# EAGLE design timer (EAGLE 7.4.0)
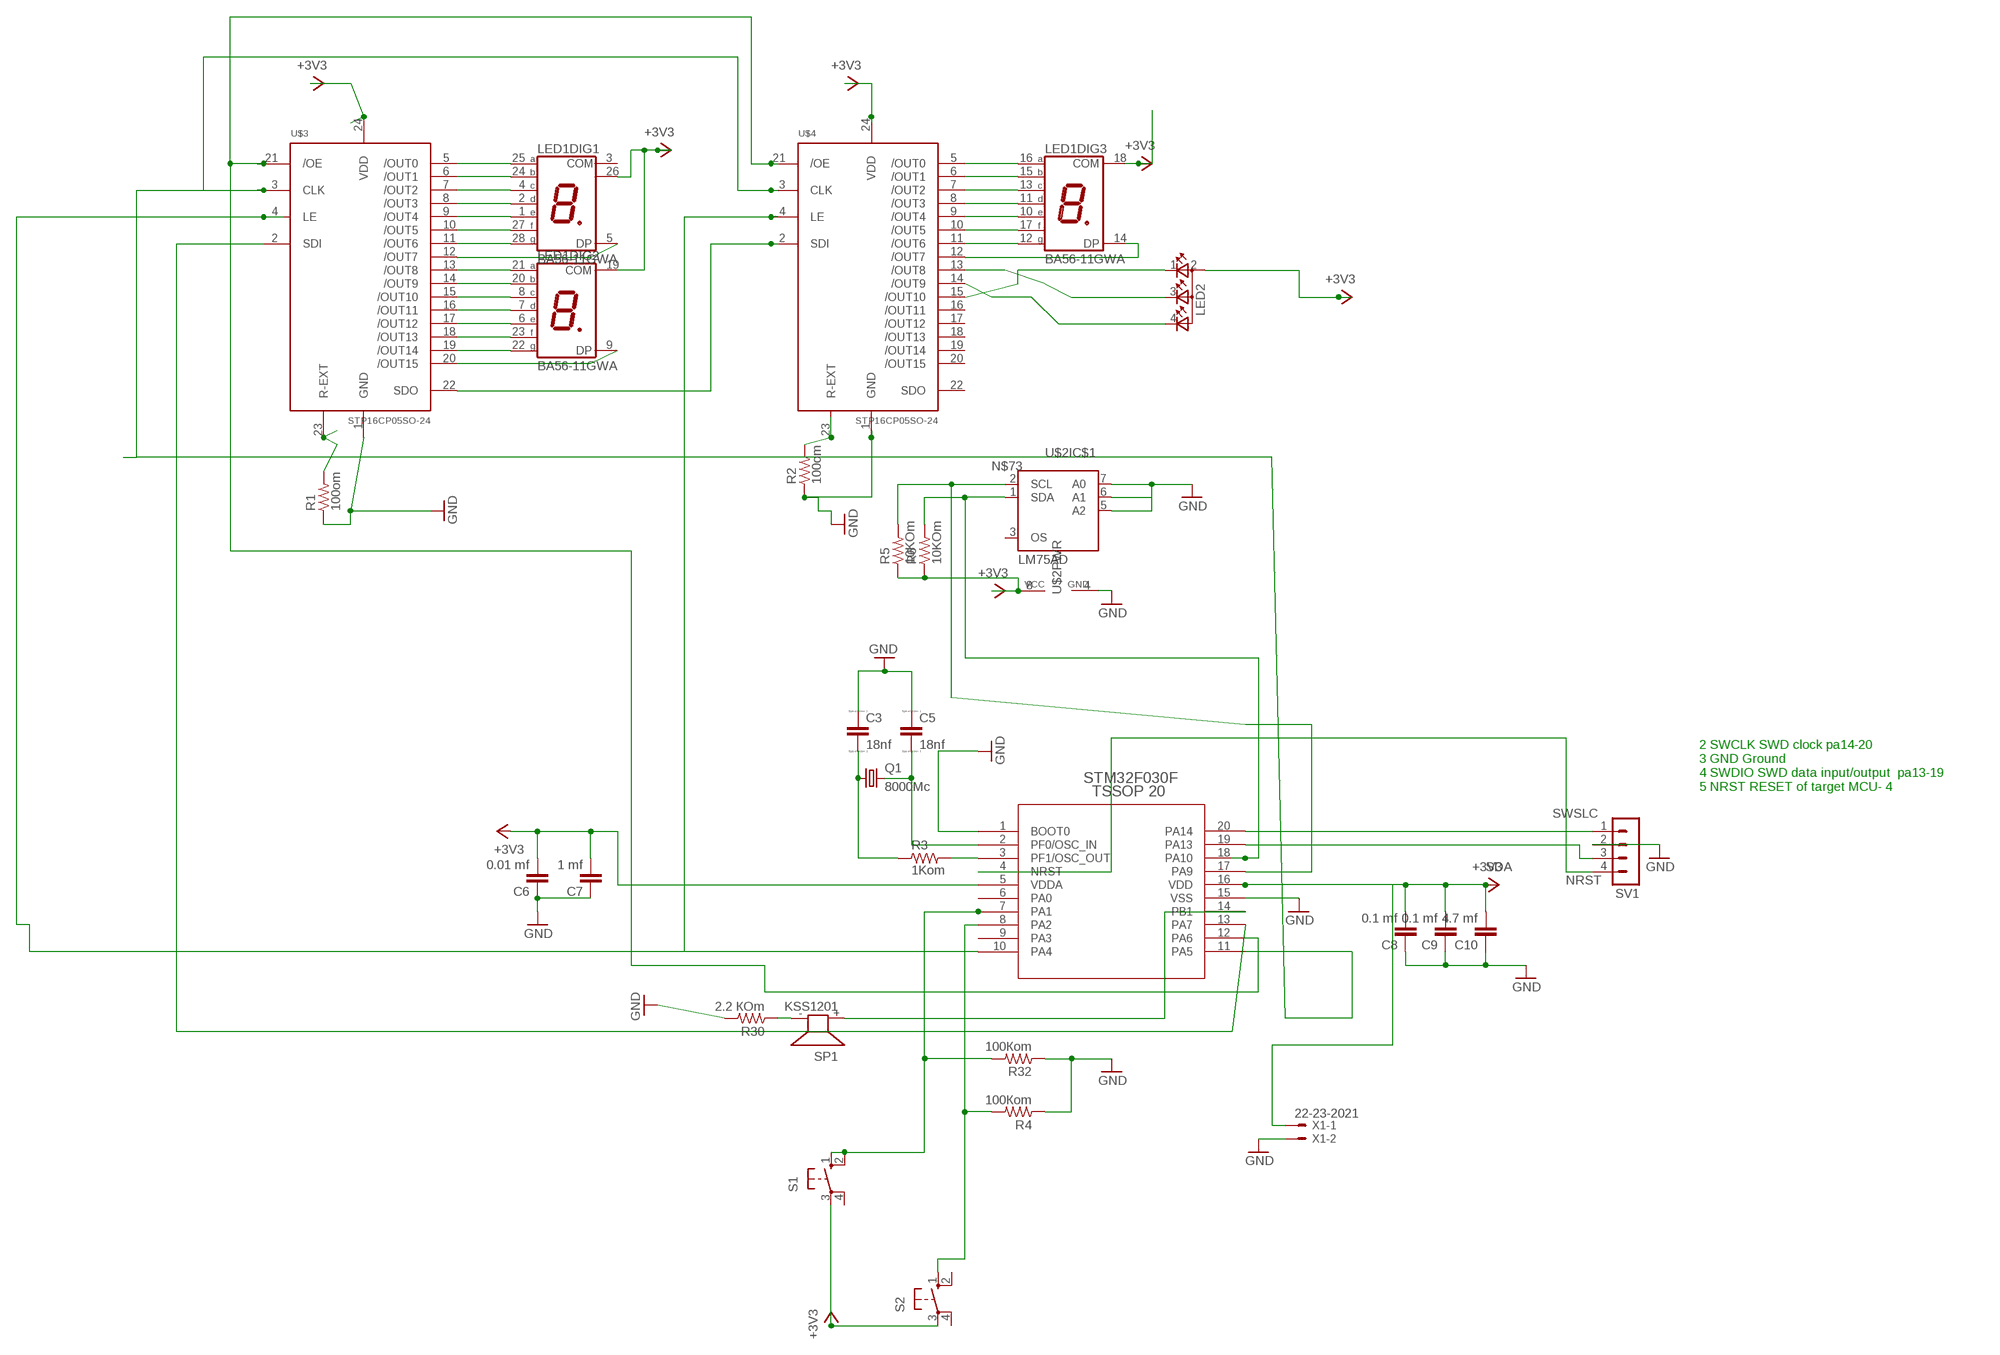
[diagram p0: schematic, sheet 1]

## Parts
C3  18nf  CC1206  [C1206]
C5  18nf  CC1206  [C1206]
C6  0.01 mf  CAP1206  [1206]
C7  1 mf  CAP1206  [1206]
C8  0.1 mf  CAP1206  [1206]
C9  0.1 mf  CAP1206  [1206]
C10  4.7 mf  CAP1206  [1206]
LED1  BA56-11GWA  [BA/BC56]
LED2  TOPLED-3  [P-LCC-4-3]
Q1  8000Mc  CRYSTALHC49S  [HC49/S]
R1  100om  STM32F050F-BASE_R_1206  [STM32F050F-BASE_R1206]
R2  100om  STM32F050F-BASE_R_1206  [STM32F050F-BASE_R1206]
R3  1Kom  STM32F050F-BASE_R_1206  [STM32F050F-BASE_R1206]
R4  100Кom  STM32F050F-BASE_R_1206  [STM32F050F-BASE_R1206]
R5  10KOm  STM32F050F-BASE_R_1206  [STM32F050F-BASE_R1206]
R6  10KOm  STM32F050F-BASE_R_1206  [STM32F050F-BASE_R1206]
R30  2.2 КOm  STM32F050F-BASE_R_1206  [STM32F050F-BASE_R1206]
R32  100Кom  STM32F050F-BASE_R_1206  [STM32F050F-BASE_R1206]
S1  10-XX  [B3F-10XX]
S2  10-XX  [B3F-10XX]
SP1  KSS1201  [KSS1201]
SV1  MA04-1  [MA04-1]
U$1  STM32F030F  [STM32F050F-BASE_TSSOP20]
U$2  LM75AD  [SO08]
U$3  STP16CP05SO-24  [SO-24]
U$4  STP16CP05SO-24  [SO-24]
X1  22-23-2021  [22-23-2021]

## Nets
+3V3: C6.2 C7.2 C8.2 C9.2 C10.2 LED1.18(DIG3:COM) LED1.19(DIG2:COM) LED1.26(DIG1:COM) LED2.2(A2) R5.1 R6.1 S1.3(P) S2.3(P) U$1.5(VDDA) U$1.16(VDD) U$2.8(PWR:VCC) U$3.24(VDD) U$4.24(VDD) X1.1
GND: C3.1 C5.1 C6.1 C7.1 C8.1 C9.1 C10.1 R1.1 R2.1 R4.1 R30.2 R32.1 SV1.2 U$1.1(BOOT0) U$1.15(VSS) U$2.4(PWR:GND) U$2.5(IC$1:A2) U$2.6(IC$1:A1) U$2.7(IC$1:A0) U$3.1(GND) U$4.1(GND) X1.2
N$1: C5.2 Q1.2 U$1.2(PF0/OSC_IN)
N$2: C3.2 Q1.1 R3.1
N$3: LED1.27(DIG1:F) U$3.10(/OUT5)
N$4: LED1.17(DIG3:F) U$4.10(/OUT5)
N$5: LED1.11(DIG3:D) U$4.8(/OUT3)
N$6: LED1.15(DIG3:B) U$4.6(/OUT1)
N$7: LED1.16(DIG3:A) U$4.5(/OUT0)
N$8: LED1.2(DIG1:D) U$3.8(/OUT3)
N$9: LED1.24(DIG1:B) U$3.6(/OUT1)
N$10: LED1.25(DIG1:A) U$3.5(/OUT0)
N$11: LED1.4(DIG1:C) U$3.7(/OUT2)
N$12: LED1.1(DIG1:E) U$3.9(/OUT4)
N$13: LED1.28(DIG1:G) U$3.11(/OUT6)
N$14: U$1.10(PA4) U$3.4(LE) U$4.4(LE)
N$15: LED1.13(DIG3:C) U$4.7(/OUT2)
N$16: U$1.13(PA7) U$3.2(SDI)
N$17: LED1.10(DIG3:E) U$4.9(/OUT4)
N$18: LED1.12(DIG3:G) U$4.11(/OUT6)
N$19: LED2.1(CRED) U$4.15(/OUT10)
N$20: LED2.3(CBLUE) U$4.13(/OUT8)
N$21: LED2.4(CGREEN) U$4.14(/OUT9)
N$22: R6.2 U$1.18(PA10) U$2.1(IC$1:SDA)
N$23: LED1.5(DIG1:DP) U$3.12(/OUT7)
N$24: U$3.22(SDO) U$4.2(SDI)
N$25: LED1.23(DIG2:F) U$3.18(/OUT13)
N$26: R4.2 S2.1(S) U$1.8(PA2)
N$28: R30.1 SP1.-
N$29: SP1.+ U$1.14(PB1)
N$30: R3.2 U$1.3(PF1/OSC_OUT)
N$31: LED1.7(DIG2:D) U$3.16(/OUT11)
N$32: LED1.20(DIG2:B) U$3.14(/OUT9)
N$33: LED1.21(DIG2:A) U$3.13(/OUT8)
N$34: LED1.8(DIG2:C) U$3.15(/OUT10)
N$35: LED1.6(DIG2:E) U$3.17(/OUT12)
N$36: LED1.22(DIG2:G) U$3.19(/OUT14)
N$37: LED1.9(DIG2:DP) U$3.20(/OUT15)
N$41: R1.2 U$3.23(R-EXT)
N$43: R2.2 U$4.23(R-EXT)
N$53: LED1.14(DIG3:DP) U$4.12(/OUT7)
N$63: U$1.12(PA6) U$3.21(/OE) U$4.21(/OE)
N$66: R32.2 S1.1(S) S1.2(S1) U$1.7(PA1)
N$70: U$1.11(PA5) U$3.3(CLK) U$4.3(CLK)
N$73: R5.2 U$1.17(PA9) U$2.2(IC$1:SCL)
NRST: SV1.4 U$1.4(NRST)
SDA: SV1.3 U$1.19(PA13)
SWSLC: SV1.1 U$1.20(PA14)
Unconnected: LED1.3(DIG1:COM) S1.4(P1) S2.2(S1) S2.4(P1) U$1.6(PA0) U$1.9(PA3) U$2.3(IC$1:OS) U$4.16(/OUT11) U$4.17(/OUT12) U$4.18(/OUT13) U$4.19(/OUT14) U$4.20(/OUT15) U$4.22(SDO)

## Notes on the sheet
- 2 SWCLK SWD clock pa14-20 
  3 GND Ground 
  4 SWDIO SWD data input/output  pa13-19 
  5 NRST RESET of target MCU- 4

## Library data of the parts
C3 C5 = eagle-ltspice:C: CAPACITOR, European symbol; SPICEMODEL: NONE; SPICEPREFIX: C
C6-C10 = SparkFun-Capacitors:CAP: Capacitor
LED1 = clockclock1:B?56-11*WA: 14.22mm (0.56INCH) THREE DIGIT NUMERIC DISPLAY Source: http://www.kingbright.com .. BA56-11EWA(Ver1189474895.pdf; OC_FARNELL: unknown; OC_NEWARK: unknown
LED2 = clockclock1:TOPLED-3: OSRAM - Hyper Multi TOPLED® (RGB) LB E673, LV E673, LT E673 - Power TOPLED® Enhanced optical Power LED (HOP2000) LS E67B, LA E67B, LO E67B, LY E67B - Hyper Multi TOPLED® Enhanced optical Power LED (HOP2000 / ATON®) LATB T66B - Hyper Multi TOPLED® Hyper-Bright LED LATB T686 Source: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
Q1 = crystal:CRYSTAL: CRYSTAL; OC_FARNELL: 1667008; OC_NEWARK: unknown
R1-R6 R30 R32 = clockclock1:STM32F050F-BASE_R_: RESISTOR
S1 S2 = switch-omron:10-XX: OMRON SWITCH; MPN: B3F-1000; OC_FARNELL: 176432; OC_NEWARK: 36M3542
SP1 = buzzer:KSS1201: SPEAKER; OC_FARNELL: unknown; OC_NEWARK: unknown
SV1 = con-lstb:MA04-1: PIN HEADER; OC_FARNELL: unknown; OC_NEWARK: unknown
U$1 = clockclock1:STM32F030F: STM32F050F4P6
U$2 = i2c:LM75AD: Digital Temperature Sensor and Thermal Watchdog
U$3 U$4 = Synapseware:STP16CP05: Low voltage 16-bit constant current LED sink driver The STP16CP05 is a monolithic, low voltage, low current power 16-bit shift register designed for LED panel displays. The STP16CP05 contains a 16-bit serial-in, parallel-out shift register that feeds a 16-bit, D-type storage register. In the output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
X1 = con-molex:22-23-2021: .100" (2.54mm) Center Header - 2 Pin; MF: MOLEX; MPN: 22-23-2021; OC_FARNELL: 1462926; OC_NEWARK: 25C3832

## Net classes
0 default: width 0.254 mm, drill 0.254 mm, clearance 0.2 mm

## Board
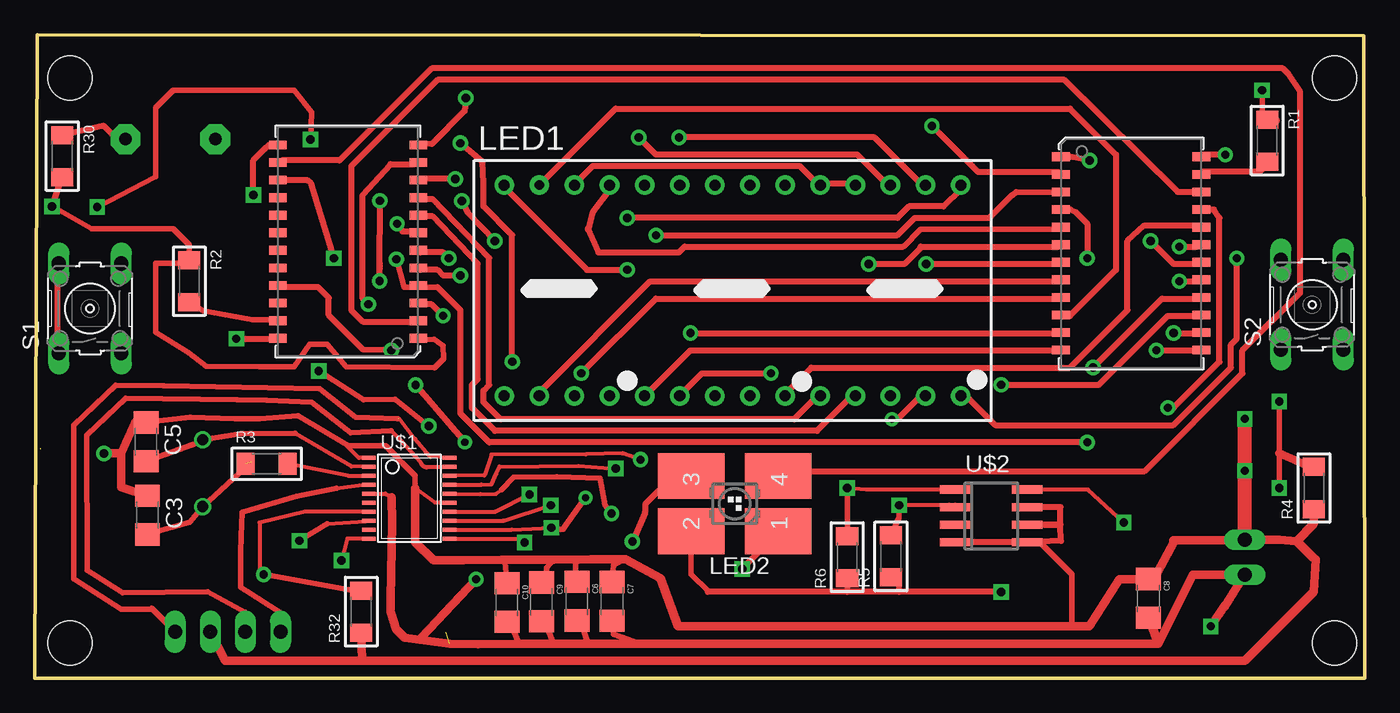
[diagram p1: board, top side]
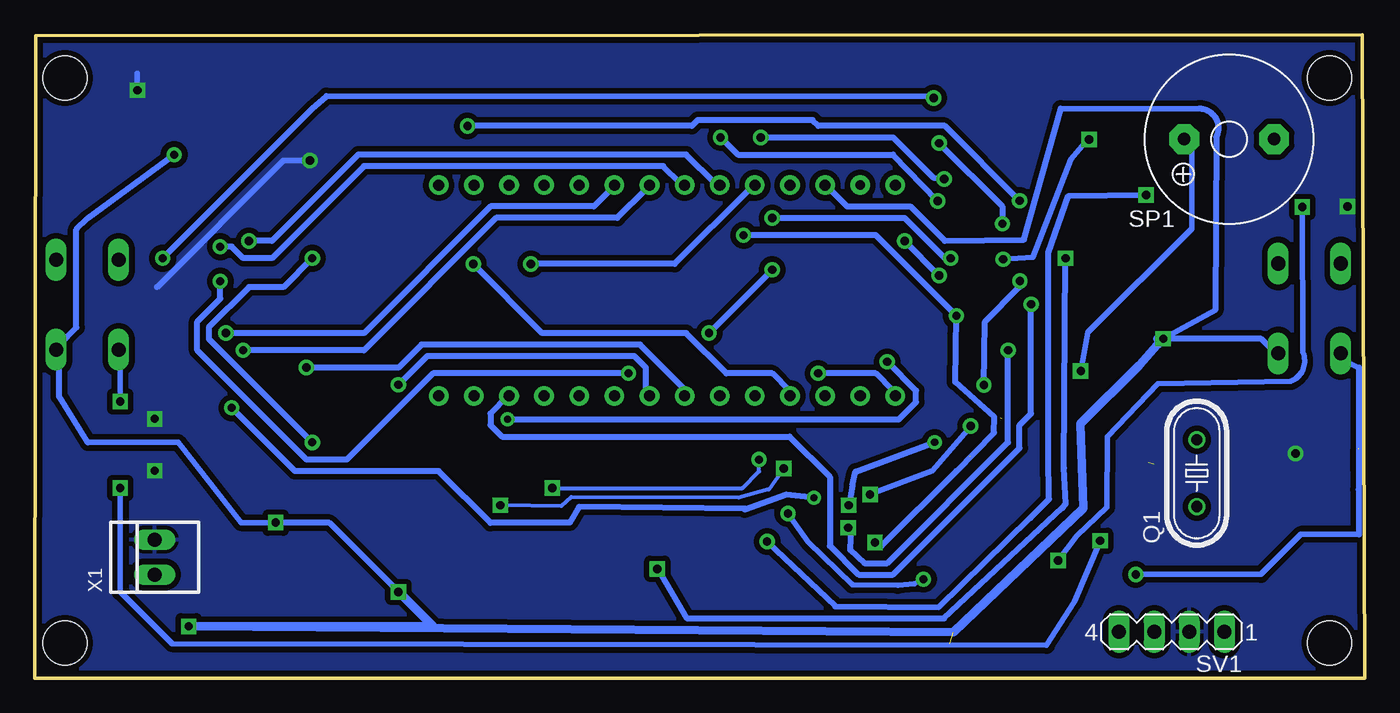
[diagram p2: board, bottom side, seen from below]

Size 96.19 x 46.53 mm. Coordinates in mm from the lower left corner, seen from the top.
Outline: 0,0 96.19,0 96.11,46.44 0.18,46.53 0,0
Copper layers (1*16): Top 0.035mm / dielectric 1.5mm / Bottom 0.035mm
Design rules "default *": minimum track width 8mil, minimum drill 10mil, track to track 4mil, track to pad 4mil, pad to pad 4mil, via to via 4mil, smd to smd 4mil, copper to edge 4mil, drill to drill 4mil, minimum pad ring 8mil, minimum via ring 8mil, stop-mask expansion 4mil, vias tented up to drill 0mil, thermal gap 10mil
Holes 3.2 mm at 2.54,43.38 2.54,2.54 93.98,2.54 93.98,43.38

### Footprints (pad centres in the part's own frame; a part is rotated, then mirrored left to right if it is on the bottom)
C1206 = smd 1.6 x 1.8: 1 -1.4,0; 2 1.4,0
1206 = smd 1.6 x 1.8: 1 -1.4,0; 2 1.4,0
BA/BC56 = drill 0.8 pad 1.422: 1 -16.51,-7.62; 2 -13.97,-7.62; 3 -11.43,-7.62; 4 -8.89,-7.62; 5 -6.35,-7.62; 6 -3.81,-7.62; 7 -1.27,-7.62; 8 1.27,-7.62; 9 3.81,-7.62; 10 6.35,-7.62; 11 8.89,-7.62; 12 11.43,-7.62; 13 13.97,-7.62; 14 16.51,-7.62; 15 16.51,7.62; 16 13.97,7.62; 17 11.43,7.62; 18 8.89,7.62; 19 6.35,7.62; 20 3.81,7.62; 21 1.27,7.62; 22 -1.27,7.62; 23 -3.81,7.62; 24 -6.35,7.62; 25 -8.89,7.62; 26 -11.43,7.62; 28 -16.51,7.62 | drill 0.7 pad 1.422: 27 -13.97,7.62
P-LCC-4-3 = smd 3.3 x 4.8: 1 -2,-3.15; 2 -2,3.15; 3 2,3.15; 4 2,-3.15
HC49/S = drill 0.813: 1 -2.413,0; 2 2.413,0
STM32F050F-BASE_R1206 = smd 1.3 x 1.6: 1 -1.524,0; 2 1.524,0
B3F-10XX = drill 1.016 long: 1 -3.251,2.261; 2 3.251,2.261; 3 -3.251,-2.261; 4 3.251,-2.261
KSS1201 = drill 0.914 pad 2.159 octagon: + 3.251,0; - -3.251,0
MA04-1 = drill 1.016 long: 1 -3.81,0; 2 -1.27,0; 3 1.27,0; 4 3.81,0
STM32F050F-BASE_TSSOP20 = smd 0.305 x 0.991: 1 -2.925,-2.918; 2 -2.275,-2.918; 3 -1.625,-2.918; 4 -0.975,-2.918; 5 -0.325,-2.918; 6 0.325,-2.918; 7 0.975,-2.918; 8 1.625,-2.918; 9 2.275,-2.918; 10 2.925,-2.918; 11 2.925,2.918; 12 2.275,2.918; 13 1.625,2.918; 14 0.975,2.918; 15 0.325,2.918; 16 -0.325,2.918; 17 -0.975,2.918; 18 -1.625,2.918; 19 -2.275,2.918; 20 -2.925,2.918
SO08 = smd 0.6 x 2.2: 1 -1.905,-2.6; 2 -0.635,-2.6; 3 0.635,-2.6; 4 1.905,-2.6; 5 1.905,2.6; 6 0.635,2.6; 7 -0.635,2.6; 8 -1.905,2.6
SO-24 = smd 1.27 x 0.635: 1 -5.08,7.62; 2 -5.08,6.35; 3 -5.08,5.08; 4 -5.08,3.81; 5 -5.08,2.54; 6 -5.08,1.27; 7 -5.08,0; 8 -5.08,-1.27; 9 -5.08,-2.54; 10 -5.08,-3.81; 11 -5.08,-5.08; 12 -5.08,-6.35; 13 5.08,-6.35; 14 5.08,-5.08; 15 5.08,-3.81; 16 5.08,-2.54; 17 5.08,-1.27; 18 5.08,0; 19 5.08,1.27; 20 5.08,2.54; 21 5.08,3.81; 22 5.08,5.08; 23 5.08,6.35; 24 5.08,7.62
22-23-2021 = drill 1 long: 1 -1.27,0; 2 1.27,0

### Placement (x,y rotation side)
C3  8.14,11.79 270 top
C5  8.04,17.09 270 top
C6  39.2,5.57 270 top
C7  41.75,5.56 270 top
C8  80.53,5.77 270 top
C9  36.63,5.52 270 top
C10  34.14,5.47 270 top
LED1  50.45,28.03 0 top
LED2  50.62,12.62 90 top
Q1  12.14,14.82 90 bottom
R1  89.12,38.86 270 top
R2  11.17,28.7 270 top
R3  16.77,15.5 0 top
R4  92.5,13.75 90 top
R5  61.91,8.81 90 top
R6  58.75,8.75 90 top
R30  1.98,37.74 270 top
R32  23.6,4.81 90 top
S1  3.99,26.73 90 top
S2  92.37,27 90 top
SP1  9.8,38.97 180 bottom
SV1  13.95,3.36 180 bottom
U$1  27.08,13.01 270 top
U$2  69.17,11.73 270 top
U$3  79.28,30.07 0 top
U$4  22.65,32.2 180 top
X1  87.5,8.75 90 bottom

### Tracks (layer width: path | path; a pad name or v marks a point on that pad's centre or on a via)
+3V3  (via drill 0.6, 0.6 pad 0.61)  (1 unrouted)
  Top 0.305: v78.75,11.25 76.16,13.63 U$2.8 | 48.71,6.29 48.75,6.25 | U$1.5 25.34,13.35 25.8,13.09 | U$1.16 32.2,13.3 33.32,13.32 33.77,13.64 | 26.73,2.94 27.92,2.94
  Top 0.406: C10.2 34.16,4.59 35,2.5 | C9.2 36.72,4.53 37.5,2.5 | C6.2 39.4,4.35 40,2.5 | C7.2 41.84,3.16 43.75,2.5 | LED2.2 47.47,7.53 48.71,6.29 | 33.77,13.64 34.62,14.52 37.74,14.56 40.89,14.45 41.25,12.5 v41.71,11.9 | R5.1 62.5,7.29 62.5,6.24 | R6.1 58.75,6.24
  Top 0.432: v14.57,24.54 17.47,24.54 U$4.24 | LED1.26 39.09,35.77 40.34,37.02 55.31,37.02 56.56,35.77 LED1.19 56.98,35.77 59.06,35.77 LED1.18 | v86.09,37.85 84.43,37.85 U$3.24 | v69.87,6.24 62.5,6.24 58.75,6.24 48.66,6.24 48.71,6.29
  Top 0.61: X1.1 83.73,7.48 81.25,2.5 | 81.25,2.5 43.75,2.5 40,2.5 37.5,2.5 35,2.5 32.06,2.47 30,2.5 26.73,2.94 26.12,3.55 25.74,4.8 25.72,5.71 25.82,11.24 25.8,13.09 | C8.2 80.53,4.47 81.25,2.5 | 86.11,5.31 v85.04,3.75 | 27.92,2.94 v31.91,7.16
  Bottom 0.406: 92.33,17.05 85.8,17.05 81.25,11.25 v78.75,11.25 | v31.91,7.16 32.56,6.83 33.76,6.72 37.06,6.74 | 37.06,6.81 37.06,6.74 | 37.06,6.74 40.26,9.88 v41.71,11.9
  Bottom 0.432: S1.3 6.65,23.71 7.49,24.54 v14.57,24.54 10.82,26.61 10.74,39.12 arc-116 11.96,41.19 21.97,41.17 24.64,31.7 30.36,31.61 32.86,34.1 37.43,34.1 38.68,35.35 LED1.26 | v86.09,37.85 92.34,33.27 93.16,32.45 93.16,25.37 94.41,24.12 S2.3 94.41,23.71 94.41,20.38 92.33,17.05 | v69.87,6.24 74.86,11.22 v78.75,11.25 | 87.75,7.49 X1.1
  Bottom 0.61: 15,24.54 v14.57,24.54 15,24.1 16.29,22.62 20.56,18.4 20.36,12.27 29.74,3.33 v85.04,3.75 67.36,3.75 v69.87,6.24
GND  (via drill 0.6)  (1 unrouted)
  Top 0.305: 33.98,7.35 C10.1 | 27.88,24.43 U$4.1 | U$1.1 23.43,15.94 22.5,16.86 22.96,16.81 | C5.1 7.24,18.49 | 23.67,1.33 23.75,1.25 | U$1.15 28.93,12.69 27.5,13.75 | 27.5,14.65 27.49,14.65
  Top 0.406: C9.1 37.01,7.17 37.01,7.99 37.5,8.57 | C6.1 39.09,7.17 39.09,8.41 40.2,8.61 | U$2.5 72.67,9.82 75,7.5 75,3.75 | 82.41,9.91 83.75,10 | 87.48,10 X1.2 | 27.88,24.43 28.88,24.51 29.53,24.05 29.57,23.1 28.92,22.46 22.5,22.5 21.13,24.16 19.88,24.16 18.75,22.5 16.25,22.5 12.38,22.54 11.12,23.52 8.75,25 8.75,30 10.95,30 R2.1 11.17,31.33 10,32.5 4.1,32.5 v1.25,34.1 | C5.1 11.23,18.86 14.47,18.77 16.25,18.75 19.03,18.99 22.62,16.84 22.96,16.81 23.76,16.81 25.36,16.8 26.07,16.08 26.62,15.52 | 26.62,15.52 26.64,15.53 | 33.75,8.57 33.99,8.39 C10.1 | C7.1 41.84,8.16 42.7,8.61 | 27.5,13.75 27.5,14.65 | 27.49,14.65 26.62,15.52 | R1.1 88.75,40.38 v88.75,42.5
  Top 0.432: C9.1 37.01,7.07 37.01,7.17 | 39.09,7.17 39.09,7.07 C6.1 | U$2.4 67.06,9.84 71.64,9.84 U$2.5 74.2,9.92 74.16,11.02 U$2.6 74.18,11.13 74.18,12.38 U$2.7 | v1.25,34.1 R30.2 | v76.27,37.43 74.89,37.68 U$3.1 | 89.84,40.31 89.42,40.34 R1.1 | 82.35,9.98 82.41,9.91 | 87.34,9.98 X1.2
  Top 0.61: 82.41,9.91 80.92,7.17 C8.1 78.42,7.17 76.25,3.75 75,3.75 46.51,3.75 45.26,7.24 42.7,8.61 40.2,8.61 37.5,8.57 33.75,8.57 31.02,8.52 28.82,8.52 27.5,9.84 27.5,13.75 | 87.48,10 90,10 91.25,9.91 | 92.63,8.62 92.5,6.25 87.5,1.25 23.75,1.25 13.75,1.25 SV1.2 | 87.34,9.98 82.35,9.98 | 7.24,18.49 6.25,16.25 | 6.25,16.25 6.25,13.8 C3.1 | R32.1 23.67,1.33 | v5,16.25 6.25,16.25 | 92.5,8.67 91.25,9.91 | R4.1 92.5,11.17 91.25,9.91
  Top 1.016: X1.2 v87.5,15 v87.5,18.75
  Bottom 0.406: v88.75,42.5 88.75,43.75
  Bottom 0.432: v76.27,37.43 78.19,37.43 87.34,28.28
  pour Bottom (isolate 0.406): 0,46.25 0,0 96.25,0 96.25,46.25
N$1
  Top 0.305: U$1.2 22.89,15.31 18.82,17.71
  Top 0.406: 18.82,17.71 14.88,17.68 Q1.2 12.28,17.21 C5.2
N$2  (1 unrouted)
  Top 0.406: C3.2 11.21,11.28 Q1.1 15.63,15.62
N$3
  Top 0.432: U$3.10 74.45,26.2 74.86,26.2 78.19,29.53 78.19,37.85 74.86,41.17 42.01,41.17 36.6,35.77 LED1.27
N$4  (via drill 0.6)
  Top 0.432: v30.4,36.09 27.91,36.09 U$4.10 | v43.66,39.09 44.91,37.85 59.47,37.85 61.55,35.77 LED1.17
  Bottom 0.432: v30.4,36.09 31.19,36.18 34.1,39.09 v43.66,39.09
N$5
  Top 0.432: U$4.8 27.93,33.38 28.77,33.38 32.02,29.95 32.02,21.63 31.61,21.21 31.61,19.55 33.27,17.88 56.56,17.88 59.06,20.38 LED1.11
N$6  (via drill 0.6)
  Top 0.432: v29.95,30.36 29.53,30.78 27.86,30.78 U$4.6 | v42.84,33.27 62.38,33.27 63.22,34.1 65.71,34.1 66.96,35.35 LED1.15
  Bottom 0.432: v29.95,30.36 30.36,30.36 33.27,33.27 v42.84,33.27
N$7  (via drill 0.6)
  Top 0.432: v30.78,29.11 29.53,29.11 29.11,29.53 27.86,29.53 U$4.5 | v33.27,31.61 31.31,33.69 v30.88,34.51 | v46.58,39.09 60.72,39.09 64.05,35.77 LED1.16
  Bottom 0.432: v33.27,31.61 v30.78,29.11 | v30.88,34.51 34.1,37.85 45.33,37.85 v46.58,39.09
N$8
  Top 0.432: U$3.8 74.03,28.7 44.5,28.7 36.6,20.8 LED1.2
N$9  (via drill 0.6)
  Top 0.432: v60.3,29.95 62.93,29.97 64.05,31.09 64.05,31.19 74.03,31.19 U$3.6
  Bottom 0.432: v60.3,29.95 49.91,29.95 44.5,35.35 LED1.24
N$10
  Top 0.432: U$3.5 73.63,32.49 64.05,32.44 62.8,31.19 47,31.19 46.58,30.78 40.75,30.78 40,32.5 40,32.44 40.34,33.69 41.59,35.35 LED1.25
N$11  (via drill 0.6)
  Top 0.432: v64.47,29.95 74.03,29.95 U$3.7
  Bottom 0.432: v64.47,29.95 59.47,24.95 49.08,24.95 46.16,22.04 42.84,22.04 41.59,20.8 LED1.4
N$12  (via drill 0.6)
  Top 0.432: v39.51,22.04 44.92,27.45 74.03,27.45 U$3.9
  Bottom 0.432: v39.51,22.04 35.35,22.04 34.1,20.8 LED1.1
N$13  (via drill 0.6)
  Top 0.432: v47.41,24.95 74.03,24.95 U$3.11 | v42.84,29.53 39.93,29.53 34.1,35.35 LED1.28
  Bottom 0.432: v42.84,29.53 v47.41,24.95
N$14  (via drill 0.6)
  Top 0.305: U$1.10 22.59,10.09 v22.17,8.5
  Top 0.406: v26.15,30.29 26.72,28.28 27.86,28.28 29.11,28.28 | v4.51,34.06 8.75,36.25 8.75,41.25 10,42.5 18.75,42.5 20,40.93 v19.93,38.95
  Top 0.432: 29.11,28.28 30.78,26.62 30.78,19.13 32.86,17.05 v76.11,17.05 | v76.11,30.36 76.11,32.86 75.28,33.69 74.91,33.88 U$3.4 | 27.86,28.28 U$4.4
  Bottom 0.406: v22.17,8.5 20.82,10.3 18.65,12.35 18.62,17.47 14.94,21.28 5.33,21.46 arc-90 4.46,23.56 v4.51,34.06 | v26.15,30.29 23.98,30.44 21.25,37.5 20,38.95 v19.93,38.95
  Bottom 0.432: v76.11,17.05 83.6,24.54 83.6,25.37 80.69,28.28 78.19,28.28 v76.11,30.36
N$15  (via drill 0.51, 0.6)
  Top 0.432: v26.2,32.86 26.58,32.3 27.41,32.3 U$4.7 | v30.78,38.68 32.4,37.34 32.44,35.77 32.44,34.1 34.52,32.02 v34.52,22.88 | v61.97,18.71 62.38,18.71 64.05,20.38 LED1.13
  Bottom 0.432: v26.2,32.86 26.2,34.1 v30.78,38.68 | v34.52,22.88 32.44,20.8 32.44,19.96 33.69,18.71 v61.97,18.71
N$16  (via drill 0.51, 0.6)
  Top 0.305: U$1.13 33.88,11.38 v37.31,12.5
  Top 0.432: v64.88,39.93 68.21,36.6 74.03,36.6 U$3.2 | v24.93,28.71 24.93,29.98 24.92,29.58 v24.95,34.52 | v31.1,17.07 v27.54,21.2
  Bottom 0.432: v64.88,39.93 48.66,39.93 48.24,40.34 39.93,40.34 39.51,39.93 30.36,39.93 v24.95,34.52 | v24.93,28.71 24.96,28.28 24.98,28.26 25,28.26 25.02,28.28 27.45,25.79 v27.54,21.2 | v31.1,17.07 36.82,14.93 37.03,13.95 v37.31,12.5
N$17
  Top 0.432: U$4.9 27.93,34.64 28.76,34.64 32.86,30.36 32.86,21.21 32.44,20.8 32.44,19.96 33.69,18.71 54.9,18.71 56.56,20.38 LED1.10
N$18  (via drill 0.6)
  Top 0.432: v24.12,27.03 23.71,27.45 23.71,34.94 25.72,37.16 27.38,37.16 U$4.11
  Bottom 0.432: v24.12,27.03 24.12,19.13 24.95,18.3 24.95,16.64 34.1,7.49 36.6,7.49 38.68,9.57 38.68,14.56 41.59,17.47 62.38,17.47 63.22,18.3 63.22,19.13 61.97,20.38 LED1.12
N$19  (via drill 0.6, 0.6 pad 0.61)
  Top 0.432: v21.63,30.36 19.96,35.77 19.72,36 U$4.15 | v51.16,7.9 53.65,10.4 LED2.1
  Bottom 0.432: v21.63,30.36 21.74,15.2 21.62,12.61 21.86,12.32 30.41,4.33 49.03,4.35 v51.16,7.9
N$20  (via drill 0.6, 0.6 pad 0.61)
  Top 0.432: v15.8,34.93 15.8,37.43 16.64,38.26 16.92,38.54 U$4.13 | v43.22,9.88 44.12,11.98 44.13,12.57 46.16,14.56 47.41,14.56 LED2.3
  Bottom 0.432: v15.8,34.93 21.41,34.87 22.88,30.77 22.88,16.21 22.82,12.94 24.17,11.6 30.8,5.14 38.28,5.19 v43.22,9.88
N$21
  Top 0.432: U$4.14 17.88,37.43 22.04,37.43 28.7,44.09 90.26,44.09 90.67,43.68 91.5,42.43 91.5,37.43 91.5,27.86 87.34,23.71 87.34,22.04 80.27,14.97 54.07,14.97 LED2.4
N$22  (via drill 0.6)
  Top 0.305: U$2.1 60.12,13.63 v58.75,13.75 | v43.8,15.8 42.5,16.25 39.83,16.18 33.02,16.16 32.52,14.66 U$1.18
  Top 0.406: R6.2 v58.75,13.75
  Bottom 0.305: v58.75,13.75 45,13.75 43.79,14.96 v43.8,15.8
N$23
  Top 0.432: U$3.12 74.03,23.71 47.41,23.71 44.5,20.8 LED1.5
N$24
  Top 0.432: U$4.2 27.45,25.79 23.71,25.79 22.88,26.62 22.88,37.02 29.11,43.26 74.44,43.26 82.65,35.17 U$3.22
N$25  (via drill 0.6)
  Top 0.432: v80.69,31.61 82.35,29.95 84.01,29.95 U$3.18
  Bottom 0.432: v80.69,31.61 79.02,31.61 72.78,37.85 49.08,37.85 47,35.77 LED1.23
N$26  (via drill 0.6)
  Top 0.305: 21.14,11.18 23.95,11.36 U$1.8 | R4.2 92.23,15.27
  Top 0.406: v90,20 90,16.25 v90,13.75 | v19.13,9.94 21.14,11.18
  Top 0.61: 92.23,15.27 90,16.25
  Bottom 0.406: v90,13.75 90,6.25 86.25,2.5 23,2.38 21,5.51 v19.13,9.94 | v90,20 90,23.64 S2.1
N$27
  Top 0.61: 86.02,5.14 87.5,7.5
N$28
  Top 0.432: R30.1 5,39.93 6.24,38.68 SP1.-
N$29  (via drill 0.6)
  Top 0.305: U$1.14 33.28,12.04 v35.77,13.29
  Top 0.406: v28.49,18.23 26.05,20.18 23.76,20.14 v20.53,22.22
  Bottom 0.406: v35.77,13.29 31.25,15 v28.49,18.23 | v20.53,22.22 20,25 12.5,32.5 12.5,38.42 SP1.+
N$30
  Top 0.305: R3.2 22.64,14.64 U$1.3
N$31  (via drill 0.6)
  Top 0.432: v76.53,22.46 81.52,27.45 84.01,27.45 U$3.16
  Bottom 0.432: v76.53,22.46 69.87,22.46 68.21,24.12 52.4,24.12 49.08,20.8 LED1.7
N$32  (via drill 0.6)
  Top 0.432: v82.35,24.95 84.01,24.95 U$3.14
  Bottom 0.432: v82.35,24.95 72.37,24.95 63.22,34.1 55.73,34.1 54.48,35.35 LED1.20
N$33  (via drill 0.6)
  Top 0.432: v81.1,23.71 84.01,23.71 U$3.13
  Bottom 0.432: v81.1,23.71 72.37,23.71 62.8,33.27 54.07,33.27 51.99,35.35 LED1.21
N$34  (via drill 0.6)
  Top 0.432: v69.87,21.21 76.94,21.21 81.93,26.2 84.01,26.2 U$3.15
  Bottom 0.432: v69.87,21.21 67.79,23.29 52.82,23.29 51.99,22.46 51.99,20.8 LED1.8
N$35  (via drill 0.6)
  Top 0.432: v82.76,28.7 84.01,28.7 U$3.17 | v53.23,22.04 48.24,22.04 47,20.8 LED1.6
  Bottom 0.432: v82.76,28.7 82.76,27.45 84.43,25.79 84.43,23.71 76.53,15.8 73.61,15.8 67.38,22.04 v53.23,22.04
N$36  (via drill 0.6)
  Top 0.432: v82.76,31.19 84.01,31.19 U$3.19
  Bottom 0.432: v82.76,31.19 81.93,31.19 81.1,30.36 79.02,30.36 72.37,37.02 50.74,37.02 49.49,35.77 LED1.22
N$37
  Top 0.432: U$3.20 83.67,32.74 80.25,32.74 79.02,31.61 79.02,26.62 74.86,22.46 56.15,22.46 54.48,20.8 LED1.9
N$41
  Top 0.432: U$3.23 84.43,36.6 88.59,36.6 89,37.02 R1.2
N$43
  Top 0.406: R2.2 12.18,26.57 15.74,25.93 16.94,25.91 U$4.23
  Top 0.432: 17.88,25.79 U$4.23
N$53  (via drill 0.6)
  Top 0.432: v31.18,41.95 31.09,41.01 28.71,38.63 U$4.12 | v86.92,30.36 86.92,24.54 86.51,24.12 86.51,22.46 82.35,18.3 69.45,18.3 67.38,20.38 LED1.14
  Bottom 0.432: v31.18,41.95 31.32,42.11 75.08,42.07 76.11,41.17 v86.92,30.36
N$63  (via drill 0.51, 0.6)
  Top 0.305: U$1.12 34.48,10.73 v37.35,10.88 37.18,10.78
  Top 0.406: 37.18,10.78 38.2,10.78
  Top 0.432: v25.79,23.71 23.75,23.75 21.25,26.25 21.25,27.5 20.47,28.28 17.88,28.28 U$4.21 | v81.93,19.55 82.35,19.55 85.67,22.88 85.67,33.27 85.28,33.88 84.45,33.88 U$3.21 | 38.2,10.78 v39.82,13.04
  Bottom 0.432: v25.79,23.71 25.79,17.05 34.52,8.32 36.18,8.32 37.22,9.28 37.16,10.9 v37.35,10.88 | v81.93,19.55 77.36,14.97 66.96,14.97 63.22,11.23 57.5,11.25 56.83,12.38 44.74,12.25 44.83,12.19 41.82,13.27 v39.82,13.04
N$66  (via drill 0.6)  (1 unrouted)
  Top 0.305: 23.67,6.19 R32.2 | U$1.7 19.54,12.04 16.25,11.25 16.25,7.5 v16.55,7.5
  Top 0.406: v16.55,7.5 23.52,6.25 R32.2
  Top 0.432: S1.2 1.66,29.95 1.66,23.71 S1.1
  Bottom 0.406: 0.41,14.97 0.41,16.55 | 0.41,10.4 4.6,10.4 7.5,7.5 v16.55,7.5
  Bottom 0.432: 0.43,13.64 0.41,16.64 0.41,22.46 2.08,23.29 S1.1 | 0.41,10.4 0.41,11.23 0.41,12.48 0.41,14.97
N$70  (via drill 0.6)
  Top 0.305: U$1.11 34.91,10.09 35.38,9.88 v35.42,9.81
  Top 0.432: v29.53,26.2 28.7,27.03 27.86,27.03 U$4.3 | v44.92,32.02 62.38,32.02 63.63,33.27 69.04,33.27 70.71,34.94 70.95,35.15 U$3.3
  Bottom 0.432: v35.42,9.81 34.94,9.57 29.53,14.97 26.8,17.76 26.78,18.9 29.6,21.43 v29.53,26.2 35.35,32.02 v44.92,32.02
N$73  (via drill 0.6)
  Top 0.305: U$1.17 32.29,13.99 33.02,14.01 33.36,14.77 33.6,15.3 39.31,15.35 v42.02,15.15 | 66.25,12.5 66.13,12.5 v62.5,12.5
  Top 0.406: R5.2 62.5,11.58 v62.5,12.5
  Top 0.432: U$2.2 66.54,12.48 66.13,12.48 66.13,12.5
  Bottom 0.305: v42.02,15.15 43.09,13.66 45.27,13.06 57.39,13.1 58.11,12.44 v62.5,12.5
NRST
  Top 0.305: 21.84,13.73 23.69,13.98 U$1.4
  Top 0.406: SV1.4 17.76,4.74 14.88,6.59 14.88,9.09 14.92,10.27 15.01,12.01 18.93,13.16 21.84,13.73
SDA
  Top 0.305: U$1.19 30.08,15.27 28.48,15.27 arc-90 27.92,15.56 26.44,17.2 25.75,17.88
  Top 0.406: SV1.3 15.22,4.78 12.5,6.25 6.34,6.18 3.78,7.82 3.74,17.56 6.58,20.24 14.63,20.12 16.78,20.1 20.03,19.96 22.84,17.76 25.75,17.88
SWSLC  (2 unrouted)
  Top 0.305: U$1.20 arc-90 U$1.20 28.59,16.01 | 28.56,16.03 27.5,17.28 26.34,18.78
  Top 0.406: 26.25,18.75 23.2,18.86 20.59,20.91 9.33,21.16 5.84,21.18 2.8,18.28 2.8,7.2 6.25,5 8.41,5 8.45,5.04 8.46,5.04 SV1.1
